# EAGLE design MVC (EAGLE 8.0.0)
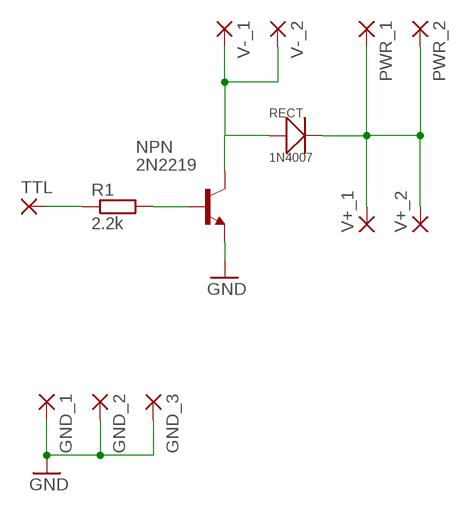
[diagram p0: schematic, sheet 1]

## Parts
GND_1  WIREPAD2,54/1,1  [2,54/1,1]
GND_2  WIREPAD2,54/1,1  [2,54/1,1]
GND_3  WIREPAD2,54/1,1  [2,54/1,1]
NPN  2N2219  [TO5]
PWR_1  WIREPAD2,54/1,1  [2,54/1,1]
PWR_2  WIREPAD2,54/1,1  [2,54/1,1]
R1  2.2k  R-EU_0309/12  [0309/12]
RECT  1N4007  DIP-DIODE-50V-1A-1N4001(DO-41)  [DO-41]
TTL  WIREPAD2,54/1,1  [2,54/1,1]
V+_1  WIREPAD2,54/1,1  [2,54/1,1]
V+_2  WIREPAD2,54/1,1  [2,54/1,1]
V-_1  WIREPAD2,54/1,1  [2,54/1,1]
V-_2  WIREPAD2,54/1,1  [2,54/1,1]

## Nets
GND: GND_1.1(P) GND_2.1(P) GND_3.1(P) NPN.1(E)
N$1: NPN.2(B) R1.2
N$2: R1.1 TTL.1(P)
N$4: PWR_1.1(P) PWR_2.1(P) RECT.2(-) V+_1.1(P) V+_2.1(P)
N$5: NPN.3(C) RECT.1(+) V-_1.1(P) V-_2.1(P)

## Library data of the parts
GND_1-GND_3 PWR_1 PWR_2 TTL V+_1 V+_2 V-_1 V-_2 = wirepad:WIREPAD: Wire PAD connect wire on PCB
NPN = transistor-npn:2N2219: NPN Transistor
R1 = resistor:R-EU_: RESISTOR, European symbol
RECT = Seeed-OPL-Diode:DIP-DIODE-50V-1A-1N4001(DO-41): 304010006; MPN: 1N4001; VALUE: 1N4001

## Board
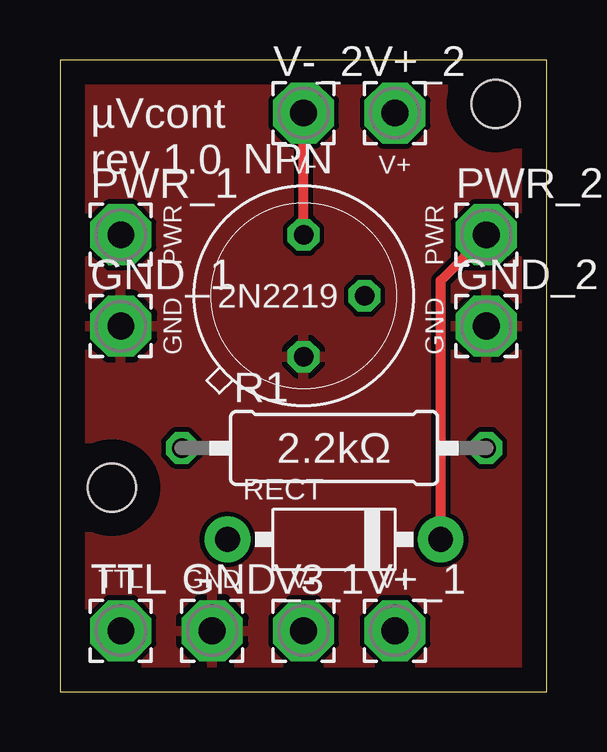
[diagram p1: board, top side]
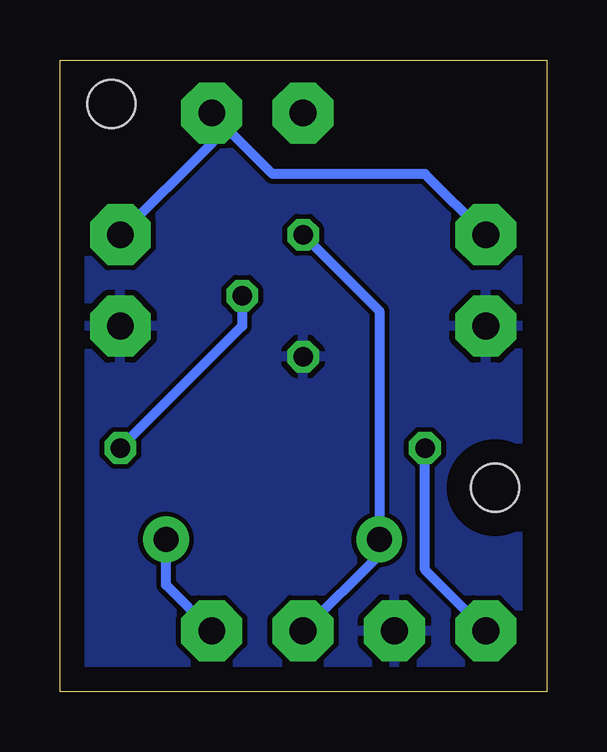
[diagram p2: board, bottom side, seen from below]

Size 20.3 x 26.34 mm. Coordinates in mm from the lower left corner, seen from the top.
Outline: 0,0 20.3,0 20.3,26.34 0,26.34 0,0
Copper layers (1*16): Top 0.035mm / dielectric 1.5mm / Bottom 0.035mm
Design rules "default": minimum track width 10mil, minimum drill 24mil, track to track 8mil, track to pad 8mil, pad to pad 8mil, via to via 8mil, smd to smd 8mil, copper to edge 40mil, drill to drill 8mil, minimum pad ring 10mil, minimum via ring 8mil, stop-mask expansion 4mil, vias tented up to drill 0mil, thermal gap 10mil
Holes 2 mm at 2.16,8.51 18.16,24.51

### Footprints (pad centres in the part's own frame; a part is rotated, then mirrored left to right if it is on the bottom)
2,54/1,1 = drill 1.118 pad 2.54 octagon: 1 0,0
TO5 = drill 0.813 octagon: 1 0,-2.54; 2 2.54,0; 3 0,2.54
0309/12 = drill 0.813 octagon: 1 -6.35,0; 2 6.35,0
DO-41 = drill 1.041 pad 1.905: 1 -4.445,0; 2 4.445,0

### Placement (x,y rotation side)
GND_1  2.54,15.24 0 top
GND_2  17.78,15.24 0 top
GND_3  6.35,2.54 0 top
NPN  10.16,16.51 0 top
PWR_1  2.54,19.05 0 top
PWR_2  17.78,19.05 0 top
R1  11.43,10.16 0 top
RECT  11.43,6.35 0 top
TTL  2.54,2.54 0 top
V+_1  13.97,2.54 0 top
V+_2  13.97,24.13 0 top
V-_1  10.16,2.54 0 top
V-_2  10.16,24.13 0 top

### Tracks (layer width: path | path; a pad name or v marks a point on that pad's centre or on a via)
GND
  pour Top: -1.27,27.94 -1.27,-1.27 21.59,-1.27 21.59,27.94
  pour Bottom: -1.27,27.94 -1.27,-1.27 21.59,-1.27 21.59,27.94
N$1
  Bottom 0.406: NPN.2 12.7,15.24 R1.2
N$2
  Bottom 0.406: TTL.1 5.08,5.08 R1.1
N$4
  Top 0.406: RECT.2 15.88,17.14 PWR_2.1
  Bottom 0.406: PWR_1.1 5.08,21.59 11.43,21.59 V+_2.1 13.97,22.86 PWR_2.1 | V+_1.1 15.88,4.45 RECT.2
N$5
  Top 0.406: NPN.3 V-_2.1
  Bottom 0.406: NPN.3 6.99,15.88 RECT.1 6.99,5.71 V-_1.1

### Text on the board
tPlace: µVcont / rev 1.0 | V- | V+ | PWR | PWR | 2N2219 | GND | GND | 2.2kΩ | TTL | GND | V- | V+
